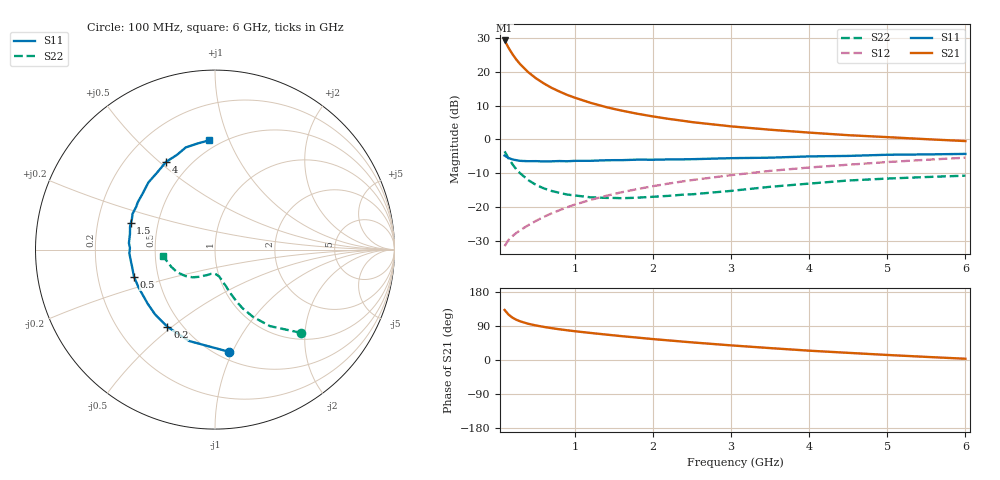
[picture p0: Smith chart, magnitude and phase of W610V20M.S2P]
! SIEMENS Small Signal Semiconductors
! BFR193W
! Si NPN RF Bipolar Junction Transistor in SOT323
! VCE = 10 V  IC = 20 mA
! Common Emitter S-Parameters:  September  1992
# GHz  S  MA  R  50
!  f  S11  S21  S12  S22
! GHz  MAG  ANG  MAG  ANG  MAG  ANG  MAG  ANG
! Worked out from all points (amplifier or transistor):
!   28 points, 100 MHz to 6 GHz, reference 50 ohm
!   highest |S21| = 29.3 dB at 100 MHz (marker M1)
!   |S21| within 3 dB of that: start of sweep to 172.2 MHz
!   unconditionally stable (mu >= 1): 824.3 MHz to 2.639 GHz
!   at 300 MHz: K = 0.73, MSG = 24.6 dB, |S12| = -26.9 dB
!   at 1.5 GHz: K = 1.04, MAG = 11.4 dB, |S12| = -16.2 dB
!   at 6 GHz: K = 0.90, MSG = 2.5 dB, |S12| = -5.4 dB
!   S11 on the Smith chart (normalised r, x): 100 MHz: 0.57, -0.97; 200 MHz: 0.42, -0.48; 500 MHz: 0.36, -0.14; 1.5 GHz: 0.35, +0.13; 4 GHz: 0.37, +0.53; 6 GHz: 0.44, +0.85
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0.1  0.5753 -82.1  29.19 132.0  0.0262 59.2  0.6666 -44.1
0.15  0.5293 -105.8  22.75 119.9  0.0324 55.3  0.5249 -54.3
0.2  0.5053 -121.6  18.33 111.8  0.0369 54.8  0.4293 -60.6
0.25  0.4916 -132.9  15.21 106.2  0.0411 55.1  0.3597 -64.9
0.3  0.481 -141.3  12.97 102.0  0.0452 56.5  0.3141 -67.4
0.4  0.4752 -153.5  9.943 95.7  0.0533 59.1  0.2504 -71.1
0.5  0.4761 -161.4  8.057 91.2  0.0619 61.6  0.2126 -73.3
0.6  0.4718 -168.1  6.768 87.4  0.071 63.3  0.1885 -75.9
0.7  0.4734 -172.8  5.813 84.1  0.08 64.6  0.1725 -77.4
0.8  0.4777 -177.5  5.124 81.1  0.0892 65.5  0.1618 -79.6
0.9  0.4741 178.9  4.565 78.5  0.0987 66.0  0.1525 -80.8
1  0.4811 175.6  4.142 75.9  0.1083 66.4  0.1477 -82.7
1.2  0.4815 169.8  3.48 71.4  0.127 66.5  0.1387 -87.1
1.5  0.4922 162.7  2.824 65.0  0.1551 66.0  0.1358 -93.4
1.8  0.5008 156.6  2.397 59.1  0.1838 65.0  0.1369 -99.2
2.2  0.5048 148.2  2.013 51.7  0.2216 62.8  0.1457 -105.6
3  0.527 134.7  1.559 38.6  0.2951 57.4  0.1727 -118.9
3.5  0.5358 127.4  1.39 31.4  0.3414 53.6  0.1985 -128.9
4  0.5596 119.2  1.26 24.6  0.3834 49.5  0.2213 -138.3
4.5  0.569 111.8  1.154 18.9  0.4215 45.5  0.246 -149.2
5.5  0.5989 99.5  1.007 8.2  0.4988 37.6  0.2769 -167.1
6  0.6093 93.2  0.944 3.3  0.5357 33.3  0.2901 -172.4
